|   stm32f427_437_429_439_lqfp176 IBIS Model
[IBIS ver]   4.2
[File name]  stm32f427_437_429_439_lqfp176.ibs
[File Rev]   1.3
[Date]   05-30-2014
[Source] Data Created at STMicroelectronics
[Notes]   File originated from ELDO simulations.
[Disclaimer]  This information is for modeling purpose only and is
   not guaranted. The information is subject to change without
   notice.
[Copyright] Copyright 2014 STMicroelectronics Inc.
[Component] stm32f427_437_429_439_lqfp176
[Manufacturer] STMicroelectronics
[Package]
| variable   typ   min   max
R_pkg   0.0   NA   NA
L_pkg   0.0H   NA   NA
C_pkg   0.0F   NA   NA
[Pin]   signal_name   model_name   R_pin   L_pin   C_pin
1   PE2   io8p_arsudq_ft   235.0E-3   11.5E-9   327.0E-15
2   PE3   io8p_arsudq_ft   229.9E-3   11.2E-9   303.3E-15
3   PE4   io8p_arsudq_ft   225.0E-3   10.8E-9   280.8E-15
4   PE5   io8p_arsudq_ft   220.4E-3   10.5E-9   259.5E-15
5   PE6   io8p_arsudq_ft   216.0E-3   10.3E-9   239.3E-15
6   VBAT   POWER   211.9E-3   10.0E-9   220.2E-15
7   PI8   io8p_arsudq_ft_v33   208.1E-3   9.7E-9   202.3E-15
8   PC13   io8p_arwsudq_ft_v33   204.4E-3   9.5E-9   185.6E-15
9   PC14   io8p_arwsudq_ft   201.1E-3   9.3E-9   170.0E-15
10   PC15   io8p_arsudq_ft   198.0E-3   9.1E-9   155.6E-15
11   PI9   io8p_arsudq_ft   195.1E-3   8.9E-9   142.3E-15
12   PI10   io8p_arsudq_ft   192.5E-3   8.7E-9   130.2E-15
13   PI11   io8p_arsudq_ft   190.1E-3   8.6E-9   119.2E-15
14   VSS   GND   188.0E-3   8.4E-9   109.4E-15
15   VDD   POWER   186.1E-3   8.3E-9   100.8E-15
16   PF0   io8p_arsudq_i2cin_ft   184.5E-3   8.2E-9   93.3E-15
17   PF1   io8p_arsudq_i2cin_ft   183.1E-3   8.1E-9   86.9E-15
18   PF2   io8p_arsudq_ft   182.0E-3   8.0E-9   81.7E-15
19   PF3   io8p_arwsudq_ft   181.1E-3   8.0E-9   77.7E-15
20   PF4   io8p_arwsudq_ft   180.5E-3   7.9E-9   74.8E-15
21   PF5   io8p_arwsudq_ft   180.1E-3   7.9E-9   73.1E-15
22   VSS   GND   180.0E-3   7.9E-9   72.5E-15
23   VDD   POWER   180.0E-3   7.9E-9   72.5E-15
24   PF6   io8p_arwsudq_ft   180.1E-3   7.9E-9   73.1E-15
25   PF7   io8p_arwsudq_ft   180.5E-3   7.9E-9   74.8E-15
26   PF8   io8p_arwsudq_ft   181.1E-3   8.0E-9   77.7E-15
27   PF9   io8p_arwsudq_ft   182.0E-3   8.0E-9   81.7E-15
28   PF10   io8p_arwsudq_ft   183.1E-3   8.1E-9   86.9E-15
29   PH0   io8p_arsudq_ft   184.5E-3   8.2E-9   93.3E-15
30   PH1   io8p_arsudq_ft   186.1E-3   8.3E-9   100.8E-15
31   NRST   ioreset_ft_v33   188.0E-3   8.4E-9   109.4E-15
32   PC0   io8p_ar3wsudq_ft   190.1E-3   8.6E-9   119.2E-15
33   PC1   io8p_ar3wsudq_ft   192.5E-3   8.7E-9   130.2E-15
34   PC2   io8p_ar3wsudq_ft   195.1E-3   8.9E-9   142.3E-15
35   PC3   io8p_ar3wsudq_ft   198.0E-3   9.1E-9   155.6E-15
36   VDD   POWER   201.1E-3   9.3E-9   170.0E-15
37   VREFM   POWER   204.4E-3   9.5E-9   185.6E-15
38   VREFP   POWER   208.1E-3   9.7E-9   202.3E-15
39   VDDA   POWER   211.9E-3   10.0E-9   220.2E-15
40   PA0   io8p_ar3wsudq_ft_v33   216.0E-3   10.3E-9   239.3E-15
41   PA1   io8p_ar3wsudq_ft   220.4E-3   10.5E-9   259.5E-15
42   PA2   io8p_ar3wsudq_ft   225.0E-3   10.8E-9   280.8E-15
43   PH2   io8p_arsudq_ft   229.9E-3   11.2E-9   303.3E-15
44   PH3   io8p_arsudq_ft   235.0E-3   11.5E-9   327.0E-15
45   PH4   io8p_arsudq_i2cin_ft   235.0E-3   11.5E-9   327.0E-15
46   PH5   io8p_arsudq_i2cin_ft   229.9E-3   11.2E-9   303.3E-15
47   PA3   io8p_ar3wsudq_ft   225.0E-3   10.8E-9   280.8E-15
48   BYPASS_REG   io8p_arsudq_ft_v33   220.4E-3   10.5E-9   259.5E-15
49   VDD   POWER   216.0E-3   10.3E-9   239.3E-15
50   PA4   io8p_ar3wsudq_ft   211.9E-3   10.0E-9   220.2E-15
51   PA5   io8p_ar3wsudq_ft   208.1E-3   9.7E-9   202.3E-15
52   PA6   io8p_ar3wsudq_ft   204.4E-3   9.5E-9   185.6E-15
53   PA7   io8p_ar3wsudq_ft   201.1E-3   9.3E-9   170.0E-15
54   PC4   io8p_ar3wsudq_ft   198.0E-3   9.1E-9   155.6E-15
55   PC5   io8p_ar3wsudq_ft   195.1E-3   8.9E-9   142.3E-15
56   PB0   io8p_ar3wsudq_ft   192.5E-3   8.7E-9   130.2E-15
57   PB1   io8p_ar3wsudq_ft   190.1E-3   8.6E-9   119.2E-15
58   PB2   io8p_ar3wsudq_ft   188.0E-3   8.4E-9   109.4E-15
59   PF11   io8p_arsudq_ft   186.1E-3   8.3E-9   100.8E-15
60   PF12   io8p_arsudq_ft   184.5E-3   8.2E-9   93.3E-15
61   VSS   GND   183.1E-3   8.1E-9   86.9E-15
62   VDD   POWER   182.0E-3   8.0E-9   81.7E-15
63   PF13   io8p_arsudq_ft   181.1E-3   8.0E-9   77.7E-15
64   PF14   io8p_arsudq_ft   180.5E-3   7.9E-9   74.8E-15
65   PF15   io8p_arsudq_ft   180.1E-3   7.9E-9   73.1E-15
66   PG0   io8p_arsudq_ft   180.0E-3   7.9E-9   72.5E-15
67   PG1   io8p_arsudq_ft   180.0E-3   7.9E-9   72.5E-15
68   PE7   io8p_arsudq_ft   180.1E-3   7.9E-9   73.1E-15
69   PE8   io8p_arsudq_ft   180.5E-3   7.9E-9   74.8E-15
70   PE9   io8p_arsudq_ft   181.1E-3   8.0E-9   77.7E-15
71   VSS   GND   182.0E-3   8.0E-9   81.7E-15
72   VDD   POWER   183.1E-3   8.1E-9   86.9E-15
73   PE10   io8p_arsudq_ft   184.5E-3   8.2E-9   93.3E-15
74   PE11   io8p_arsudq_ft   186.1E-3   8.3E-9   100.8E-15
75   PE12   io8p_arsudq_ft   188.0E-3   8.4E-9   109.4E-15
76   PE13   io8p_arsudq_ft   190.1E-3   8.6E-9   119.2E-15
77   PE14   io8p_arsudq_ft   192.5E-3   8.7E-9   130.2E-15
78   PE15   io8p_ar3wsudq_ft   195.1E-3   8.9E-9   142.3E-15
79   PB10   io8p_arsudq_i2cin_ft   198.0E-3   9.1E-9   155.6E-15
80   PB11   io8p_arsudq_i2cin_ft   201.1E-3   9.3E-9   170.0E-15
81   VCAP1   POWER   204.4E-3   9.5E-9   185.6E-15
82   VDD   POWER   208.1E-3   9.7E-9   202.3E-15
83   PH6   io8p_arsudq_ft   211.9E-3   10.0E-9   220.2E-15
84   PH7   io8p_arsudq_i2cin_ft   216.0E-3   10.3E-9   239.3E-15
85   PH8   io8p_arsudq_i2cin_ft   220.4E-3   10.5E-9   259.5E-15
86   PH9   io8p_arsudq_ft   225.0E-3   10.8E-9   280.8E-15
87   PH10   io8p_arsudq_ft   229.9E-3   11.2E-9   303.3E-15
88   PH11   io8p_arsudq_ft   235.0E-3   11.5E-9   327.0E-15
89   PH12   io8p_arsudq_ft   235.0E-3   11.5E-9   327.0E-15
90   VSS   GND   229.9E-3   11.2E-9   303.3E-15
91   VDD   POWER   225.0E-3   10.8E-9   280.8E-15
92   PB12   io8usb_id_otg_ft   220.4E-3   10.5E-9   259.5E-15
93   PB13   io8usb_vbus_otg_ft   216.0E-3   10.3E-9   239.3E-15
94   PB14   io8usb_lsfs_otg_ft   211.9E-3   10.0E-9   220.2E-15
95   PB15   io8usb_lsfs_otg_ft   208.1E-3   9.7E-9   202.3E-15
96   PD8   io8p_arsudq_ft   204.4E-3   9.5E-9   185.6E-15
97   PD9   io8p_arsudq_ft   201.1E-3   9.3E-9   170.0E-15
98   PD10   io8p_arsudq_ft   198.0E-3   9.1E-9   155.6E-15
99   PD11   io8p_arsudq_ft   195.1E-3   8.9E-9   142.3E-15
100   PD12   io8p_arsudq_ft   192.5E-3   8.7E-9   130.2E-15
101   PD13   io8p_arsudq_ft   190.1E-3   8.6E-9   119.2E-15
102   VSS   GND   188.0E-3   8.4E-9   109.4E-15
103   VDD   POWER   186.1E-3   8.3E-9   100.8E-15
104   PD14   io8p_arsudq_ft   184.5E-3   8.2E-9   93.3E-15
105   PD15   io8p_arsudq_ft   183.1E-3   8.1E-9   86.9E-15
106   PG2   io8p_arsudq_ft   182.0E-3   8.0E-9   81.7E-15
107   PG3   io8p_arsudq_ft   181.1E-3   8.0E-9   77.7E-15
108   PG4   io8p_arsudq_ft   180.5E-3   7.9E-9   74.8E-15
109   PG5   io8p_arsudq_ft   180.1E-3   7.9E-9   73.1E-15
110   PG6   io8p_arsudq_ft   180.0E-3   7.9E-9   72.5E-15
111   PG7   io8p_arsudq_ft   180.0E-3   7.9E-9   72.5E-15
112   PG8   io8p_arsudq_ft   180.1E-3   7.9E-9   73.1E-15
113   VSS   GND   180.5E-3   7.9E-9   74.8E-15
114   VDD   POWER   181.1E-3   8.0E-9   77.7E-15
115   PC6   io8p_arsudq_ft   182.0E-3   8.0E-9   81.7E-15
116   PC7   io8p_arsudq_ft   183.1E-3   8.1E-9   86.9E-15
117   PC8   io8p_arsudq_ft   184.5E-3   8.2E-9   93.3E-15
118   PC9   io8p_arsudq_i2cin_ft   186.1E-3   8.3E-9   100.8E-15
119   PA8   io8p_arsudq_i2cin_ft   188.0E-3   8.4E-9   109.4E-15
120   PA9   io8usb_vbus_otg_ft   190.1E-3   8.6E-9   119.2E-15
121   PA10   io8usb_id_otg_ft   192.5E-3   8.7E-9   130.2E-15
122   PA11   io8usb_lsfs_otg_ft   195.1E-3   8.9E-9   142.3E-15
123   PA12   io8usb_lsfs_otg_ft   198.0E-3   9.1E-9   155.6E-15
124   PA13   io8p_arsudq_ft   201.1E-3   9.3E-9   170.0E-15
125   VCAP2   POWER   204.4E-3   9.5E-9   185.6E-15
126   VSS   GND   208.1E-3   9.7E-9   202.3E-15
127   VDD   POWER   211.9E-3   10.0E-9   220.2E-15
128   PH13   io8p_arsudq_ft   216.0E-3   10.3E-9   239.3E-15
129   PH14   io8p_arsudq_ft   220.4E-3   10.5E-9   259.5E-15
130   PH15   io8p_arsudq_ft   225.0E-3   10.8E-9   280.8E-15
131   PI0   io8p_arsudq_ft   229.9E-3   11.2E-9   303.3E-15
132   PI1   io8p_arsudq_ft   235.0E-3   11.5E-9   327.0E-15
133   PI2   io8p_arsudq_ft   235.0E-3   11.5E-9   327.0E-15
134   PI3   io8p_arsudq_ft   229.9E-3   11.2E-9   303.3E-15
135   VSS   GND   225.0E-3   10.8E-9   280.8E-15
136   VDD   POWER   220.4E-3   10.5E-9   259.5E-15
137   PA14   io8p_arsudq_ft   216.0E-3   10.3E-9   239.3E-15
138   PA15   io8p_arsudq_ft   211.9E-3   10.0E-9   220.2E-15
139   PC10   io8p_arsudq_ft   208.1E-3   9.7E-9   202.3E-15
140   PC11   io8p_arsudq_ft   204.4E-3   9.5E-9   185.6E-15
141   PC12   io8p_arsudq_ft   201.1E-3   9.3E-9   170.0E-15
142   PD0   io8p_arsudq_ft   198.0E-3   9.1E-9   155.6E-15
143   PD1   io8p_arsudq_ft   195.1E-3   8.9E-9   142.3E-15
144   PD2   io8p_arsudq_ft   192.5E-3   8.7E-9   130.2E-15
145   PD3   io8p_arsudq_ft   190.1E-3   8.6E-9   119.2E-15
146   PD4   io8p_arsudq_ft   188.0E-3   8.4E-9   109.4E-15
147   PD5   io8p_arsudq_ft   186.1E-3   8.3E-9   100.8E-15
148   VSS   GND   184.5E-3   8.2E-9   93.3E-15
149   VDD   POWER   183.1E-3   8.1E-9   86.9E-15
150   PD6   io8p_arsudq_ft   182.0E-3   8.0E-9   81.7E-15
151   PD7   io8p_arsudq_ft   181.1E-3   8.0E-9   77.7E-15
152   PG9   io8p_arsudq_ft   180.5E-3   7.9E-9   74.8E-15
153   PG10   io8p_arsudq_ft   180.1E-3   7.9E-9   73.1E-15
154   PG11   io8p_arsudq_ft   180.0E-3   7.9E-9   72.5E-15
155   PG12   io8p_arsudq_ft   180.0E-3   7.9E-9   72.5E-15
156   PG13   io8p_arsudq_ft   180.1E-3   7.9E-9   73.1E-15
157   PG14   io8p_arsudq_ft   180.5E-3   7.9E-9   74.8E-15
158   VSS   GND   181.1E-3   8.0E-9   77.7E-15
159   VDD   POWER   182.0E-3   8.0E-9   81.7E-15
160   PG15   io8p_arsudq_ft   183.1E-3   8.1E-9   86.9E-15
161   PB3   io8p_arsudq_ft   184.5E-3   8.2E-9   93.3E-15
162   PB4   io8p_arsudq_ft   186.1E-3   8.3E-9   100.8E-15
163   PB5   io8p_ar3wsudq_ft   188.0E-3   8.4E-9   109.4E-15
164   PB6   io8p_arsudq_i2cin_ft   190.1E-3   8.6E-9   119.2E-15
165   PB7   io8p_arsudq_i2cin_ft   192.5E-3   8.7E-9   130.2E-15
166   BOOT0   vpp_test_hv   195.1E-3   8.9E-9   142.3E-15
167   PB8   io8p_arsudq_i2cin_ft   198.0E-3   9.1E-9   155.6E-15
168   PB9   io8p_arsudq_i2cin_ft   201.1E-3   9.3E-9   170.0E-15
169   PE0   io8p_arsudq_ft   204.4E-3   9.5E-9   185.6E-15
170   PE1   io8p_arsudq_ft   208.1E-3   9.7E-9   202.3E-15
171   PDR_ON   io8p_arsudq_ft_v33   211.9E-3   10.0E-9   220.2E-15
172   VDD_3   POWER   216.0E-3   10.3E-9   239.3E-15
173   PI4   io8p_arsudq_ft   220.4E-3   10.5E-9   259.5E-15
174   PI5   io8p_arsudq_ft   225.0E-3   10.8E-9   280.8E-15
175   PI6   io8p_arsudq_ft   229.9E-3   11.2E-9   303.3E-15
176   PI7   io8p_arsudq_ft   235.0E-3   11.5E-9   327.0E-15
[Diff Pin]   inv_pin   vdiff   tdelay_typ  tdelay_min  tdelay_max
95   94   200mV   NA   NA   NA
123   122   200mV   NA   NA   NA
[Model Selector] io8p_ar3wsudq_ft
io8p00_ar3wsudq_ft_pd_lv  "SPEED00 1P8V, PD=40kOhm"
io8p00_ar3wsudq_ft_pu_lv  "SPEED00 1P8V, PU=40kOhm"
io8p00_ar3wsudq_ft_lv  "SPEED00 1P8V"
io8p01_ar3wsudq_ft_pd_lv  "SPEED01 1P8V, PD=40kOhm"
io8p01_ar3wsudq_ft_pu_lv  "SPEED01 1P8V, PU=40kOhm"
io8p01_ar3wsudq_ft_lv  "SPEED01 1P8V"
io8p10_ar3wsudq_ft_pd_lv  "SPEED10 1P8V, PD=40kOhm"
io8p10_ar3wsudq_ft_pu_lv  "SPEED10 1P8V, PU=40kOhm"
io8p10_ar3wsudq_ft_lv  "SPEED10 1P8V"
io8p11_ar3wsudq_ft_pd_lv  "SPEED11 1P8V, PD=40kOhm"
io8p11_ar3wsudq_ft_pu_lv  "SPEED11 1P8V, PU=40kOhm"
io8p11_ar3wsudq_ft_lv  "SPEED11 1P8V"
io8p00_ar3wsudq_ft_pd  "SPEED00, PD=40kOhm"
io8p00_ar3wsudq_ft_pu  "SPEED00, PU=40kOhm"
io8p00_ar3wsudq_ft  "SPEED00"
io8p01_ar3wsudq_ft_pd  "SPEED01, PD=40kOhm"
io8p01_ar3wsudq_ft_pu  "SPEED01, PU=40kOhm"
io8p01_ar3wsudq_ft  "SPEED01"
io8p10_ar3wsudq_ft_pd  "SPEED10, PD=40kOhm"
io8p10_ar3wsudq_ft_pu  "SPEED10, PU=40kOhm"
io8p10_ar3wsudq_ft  "SPEED10"
io8p11_ar3wsudq_ft_pd  "SPEED11, PD=40kOhm"
io8p11_ar3wsudq_ft_pu  "SPEED11, PU=40kOhm"
io8p11_ar3wsudq_ft  "SPEED11"
[Model Selector] io8p_ar3wsudq_ft_v33
io8p00_ar3wsudq_ft_v33_pd_lv  "SPEED00 1P8V, PD=40kOhm"
io8p00_ar3wsudq_ft_v33_pu_lv  "SPEED00 1P8V, PU=40kOhm"
io8p00_ar3wsudq_ft_v33_lv  "SPEED00 1P8V"
io8p01_ar3wsudq_ft_v33_pd_lv  "SPEED01 1P8V, PD=40kOhm"
io8p01_ar3wsudq_ft_v33_pu_lv  "SPEED01 1P8V, PU=40kOhm"
io8p01_ar3wsudq_ft_v33_lv  "SPEED01 1P8V"
io8p10_ar3wsudq_ft_v33_pd_lv  "SPEED10 1P8V, PD=40kOhm"
io8p10_ar3wsudq_ft_v33_pu_lv  "SPEED10 1P8V, PU=40kOhm"
io8p10_ar3wsudq_ft_v33_lv  "SPEED10 1P8V"
io8p11_ar3wsudq_ft_v33_pd_lv  "SPEED11 1P8V, PD=40kOhm"
io8p11_ar3wsudq_ft_v33_pu_lv  "SPEED11 1P8V, PU=40kOhm"
io8p11_ar3wsudq_ft_v33_lv  "SPEED11 1P8V"
io8p00_ar3wsudq_ft_v33_pd  "SPEED00, PD=40kOhm"
io8p00_ar3wsudq_ft_v33_pu  "SPEED00, PU=40kOhm"
io8p00_ar3wsudq_ft_v33  "SPEED00"
io8p01_ar3wsudq_ft_v33_pd  "SPEED01, PD=40kOhm"
io8p01_ar3wsudq_ft_v33_pu  "SPEED01, PU=40kOhm"
io8p01_ar3wsudq_ft_v33  "SPEED01"
io8p10_ar3wsudq_ft_v33_pd  "SPEED10, PD=40kOhm"
io8p10_ar3wsudq_ft_v33_pu  "SPEED10, PU=40kOhm"
io8p10_ar3wsudq_ft_v33  "SPEED10"
io8p11_ar3wsudq_ft_v33_pd  "SPEED11, PD=40kOhm"
io8p11_ar3wsudq_ft_v33_pu  "SPEED11, PU=40kOhm"
io8p11_ar3wsudq_ft_v33  "SPEED11"
[Model Selector] io8p_arsudq_ft
io8p00_arsudq_ft_pd_lv  "SPEED00 1P8V, PD=40kOhm"
io8p00_arsudq_ft_pu_lv  "SPEED00 1P8V, PU=40kOhm"
io8p00_arsudq_ft_lv  "SPEED00 1P8V"
io8p01_arsudq_ft_pd_lv  "SPEED01 1P8V, PD=40kOhm"
io8p01_arsudq_ft_pu_lv  "SPEED01 1P8V, PU=40kOhm"
io8p01_arsudq_ft_lv  "SPEED01 1P8V"
io8p10_arsudq_ft_pd_lv  "SPEED10 1P8V, PD=40kOhm"
io8p10_arsudq_ft_pu_lv  "SPEED10 1P8V, PU=40kOhm"
io8p10_arsudq_ft_lv  "SPEED10 1P8V"
io8p11_arsudq_ft_pd_lv  "SPEED11 1P8V, PD=40kOhm"
io8p11_arsudq_ft_pu_lv  "SPEED11 1P8V, PU=40kOhm"
io8p11_arsudq_ft_lv  "SPEED11 1P8V"
io8p00_arsudq_ft_pd  "SPEED00, PD=40kOhm"
io8p00_arsudq_ft_pu  "SPEED00, PU=40kOhm"
io8p00_arsudq_ft  "SPEED00"
io8p01_arsudq_ft_pd  "SPEED01, PD=40kOhm"
io8p01_arsudq_ft_pu  "SPEED01, PU=40kOhm"
io8p01_arsudq_ft  "SPEED01"
io8p10_arsudq_ft_pd  "SPEED10, PD=40kOhm"
io8p10_arsudq_ft_pu  "SPEED10, PU=40kOhm"
io8p10_arsudq_ft  "SPEED10"
io8p11_arsudq_ft_pd  "SPEED11, PD=40kOhm"
io8p11_arsudq_ft_pu  "SPEED11, PU=40kOhm"
io8p11_arsudq_ft  "SPEED11"
[Model Selector] io8p_arsudq_ft_v33
io8p00_arsudq_ft_v33_pd_lv  "SPEED00 1P8V, PD=40kOhm"
io8p00_arsudq_ft_v33_pu_lv  "SPEED00 1P8V, PU=40kOhm"
io8p00_arsudq_ft_v33_lv  "SPEED00 1P8V"
io8p01_arsudq_ft_v33_pd_lv  "SPEED01 1P8V, PD=40kOhm"
io8p01_arsudq_ft_v33_pu_lv  "SPEED01 1P8V, PU=40kOhm"
io8p01_arsudq_ft_v33_lv  "SPEED01 1P8V"
io8p10_arsudq_ft_v33_pd_lv  "SPEED10 1P8V, PD=40kOhm"
io8p10_arsudq_ft_v33_pu_lv  "SPEED10 1P8V, PU=40kOhm"
io8p10_arsudq_ft_v33_lv  "SPEED10 1P8V"
io8p11_arsudq_ft_v33_pd_lv  "SPEED11 1P8V, PD=40kOhm"
io8p11_arsudq_ft_v33_pu_lv  "SPEED11 1P8V, PU=40kOhm"
io8p11_arsudq_ft_v33_lv  "SPEED11 1P8V"
io8p00_arsudq_ft_v33_pd  "SPEED00, PD=40kOhm"
io8p00_arsudq_ft_v33_pu  "SPEED00, PU=40kOhm"
io8p00_arsudq_ft_v33  "SPEED00"
io8p01_arsudq_ft_v33_pd  "SPEED01, PD=40kOhm"
io8p01_arsudq_ft_v33_pu  "SPEED01, PU=40kOhm"
io8p01_arsudq_ft_v33  "SPEED01"
io8p10_arsudq_ft_v33_pd  "SPEED10, PD=40kOhm"
io8p10_arsudq_ft_v33_pu  "SPEED10, PU=40kOhm"
io8p10_arsudq_ft_v33  "SPEED10"
io8p11_arsudq_ft_v33_pd  "SPEED11, PD=40kOhm"
io8p11_arsudq_ft_v33_pu  "SPEED11, PU=40kOhm"
io8p11_arsudq_ft_v33  "SPEED11"
[Model Selector] io8p_arsudq_i2cin_ft
io8p00_arsudq_i2cin_ft_pd_lv  "SPEED00 1P8V, PD=40kOhm"
io8p00_arsudq_i2cin_ft_pu_lv  "SPEED00 1P8V, PU=40kOhm"
io8p00_arsudq_i2cin_ft_lv  "SPEED00 1P8V"
io8p01_arsudq_i2cin_ft_pd_lv  "SPEED01 1P8V, PD=40kOhm"
io8p01_arsudq_i2cin_ft_pu_lv  "SPEED01 1P8V, PU=40kOhm"
io8p01_arsudq_i2cin_ft_lv  "SPEED01 1P8V"
io8p10_arsudq_i2cin_ft_pd_lv  "SPEED10 1P8V, PD=40kOhm"
io8p10_arsudq_i2cin_ft_pu_lv  "SPEED10 1P8V, PU=40kOhm"
io8p10_arsudq_i2cin_ft_lv  "SPEED10 1P8V"
io8p11_arsudq_i2cin_ft_pd_lv  "SPEED11 1P8V, PD=40kOhm"
io8p11_arsudq_i2cin_ft_pu_lv  "SPEED11 1P8V, PU=40kOhm"
io8p11_arsudq_i2cin_ft_lv  "SPEED11 1P8V"
io8p00_arsudq_i2cin_ft_pd  "SPEED00, PD=40kOhm"
io8p00_arsudq_i2cin_ft_pu  "SPEED00, PU=40kOhm"
io8p00_arsudq_i2cin_ft  "SPEED00"
io8p01_arsudq_i2cin_ft_pd  "SPEED01, PD=40kOhm"
io8p01_arsudq_i2cin_ft_pu  "SPEED01, PU=40kOhm"
io8p01_arsudq_i2cin_ft  "SPEED01"
io8p10_arsudq_i2cin_ft_pd  "SPEED10, PD=40kOhm"
io8p10_arsudq_i2cin_ft_pu  "SPEED10, PU=40kOhm"
io8p10_arsudq_i2cin_ft  "SPEED10"
io8p11_arsudq_i2cin_ft_pd  "SPEED11, PD=40kOhm"
io8p11_arsudq_i2cin_ft_pu  "SPEED11, PU=40kOhm"
io8p11_arsudq_i2cin_ft  "SPEED11"
[Model Selector] io8p_arwsudq_ft
io8p00_arwsudq_ft_pd_lv  "SPEED00 1P8V, PD=40kOhm"
io8p00_arwsudq_ft_pu_lv  "SPEED00 1P8V, PU=40kOhm"
io8p00_arwsudq_ft_lv  "SPEED00 1P8V"
io8p01_arwsudq_ft_pd_lv  "SPEED01 1P8V, PD=40kOhm"
io8p01_arwsudq_ft_pu_lv  "SPEED01 1P8V, PU=40kOhm"
io8p01_arwsudq_ft_lv  "SPEED01 1P8V"
io8p10_arwsudq_ft_pd_lv  "SPEED10 1P8V, PD=40kOhm"
io8p10_arwsudq_ft_pu_lv  "SPEED10 1P8V, PU=40kOhm"
io8p10_arwsudq_ft_lv  "SPEED10 1P8V"
io8p11_arwsudq_ft_pd_lv  "SPEED11 1P8V, PD=40kOhm"
io8p11_arwsudq_ft_pu_lv  "SPEED11 1P8V, PU=40kOhm"
io8p11_arwsudq_ft_lv  "SPEED11 1P8V"
io8p00_arwsudq_ft_pd  "SPEED00, PD=40kOhm"
io8p00_arwsudq_ft_pu  "SPEED00, PU=40kOhm"
io8p00_arwsudq_ft  "SPEED00"
io8p01_arwsudq_ft_pd  "SPEED01, PD=40kOhm"
io8p01_arwsudq_ft_pu  "SPEED01, PU=40kOhm"
io8p01_arwsudq_ft  "SPEED01"
io8p10_arwsudq_ft_pd  "SPEED10, PD=40kOhm"
io8p10_arwsudq_ft_pu  "SPEED10, PU=40kOhm"
io8p10_arwsudq_ft  "SPEED10"
io8p11_arwsudq_ft_pd  "SPEED11, PD=40kOhm"
io8p11_arwsudq_ft_pu  "SPEED11, PU=40kOhm"
io8p11_arwsudq_ft  "SPEED11"
[Model Selector] io8p_arwsudq_ft_v33
io8p00_arwsudq_ft_v33_pd_lv  "SPEED00 1P8V, PD=40kOhm"
io8p00_arwsudq_ft_v33_pu_lv  "SPEED00 1P8V, PU=40kOhm"
io8p00_arwsudq_ft_v33_lv  "SPEED00 1P8V"
io8p01_arwsudq_ft_v33_pd_lv  "SPEED01 1P8V, PD=40kOhm"
io8p01_arwsudq_ft_v33_pu_lv  "SPEED01 1P8V, PU=40kOhm"
io8p01_arwsudq_ft_v33_lv  "SPEED01 1P8V"
io8p10_arwsudq_ft_v33_pd_lv  "SPEED10 1P8V, PD=40kOhm"
io8p10_arwsudq_ft_v33_pu_lv  "SPEED10 1P8V, PU=40kOhm"
io8p10_arwsudq_ft_v33_lv  "SPEED10 1P8V"
io8p11_arwsudq_ft_v33_pd_lv  "SPEED11 1P8V, PD=40kOhm"
io8p11_arwsudq_ft_v33_pu_lv  "SPEED11 1P8V, PU=40kOhm"
io8p11_arwsudq_ft_v33_lv  "SPEED11 1P8V"
io8p00_arwsudq_ft_v33_pd  "SPEED00, PD=40kOhm"
io8p00_arwsudq_ft_v33_pu  "SPEED00, PU=40kOhm"
io8p00_arwsudq_ft_v33  "SPEED00"
io8p01_arwsudq_ft_v33_pd  "SPEED01, PD=40kOhm"
io8p01_arwsudq_ft_v33_pu  "SPEED01, PU=40kOhm"
io8p01_arwsudq_ft_v33  "SPEED01"
io8p10_arwsudq_ft_v33_pd  "SPEED10, PD=40kOhm"
io8p10_arwsudq_ft_v33_pu  "SPEED10, PU=40kOhm"
io8p10_arwsudq_ft_v33  "SPEED10"
io8p11_arwsudq_ft_v33_pd  "SPEED11, PD=40kOhm"
io8p11_arwsudq_ft_v33_pu  "SPEED11, PU=40kOhm"
io8p11_arwsudq_ft_v33  "SPEED11"
[Model Selector] io8usb_id_otg_ft
io8p00_id_otg_ft_pd_lv  "SPEED00 1P8V, PD=14kOhm"
io8p00_id_otg_ft_pu_lv  "SPEED00 1P8V, PU=14kOhm"
io8p00_id_otg_ft_lv  "SPEED00 1P8V"
io8p01_id_otg_ft_pd_lv  "SPEED01 1P8V, PD=14kOhm"
io8p01_id_otg_ft_pu_lv  "SPEED01 1P8V, PU=14kOhm"
io8p01_id_otg_ft_lv  "SPEED01 1P8V"
io8p10_id_otg_ft_pd_lv  "SPEED10 1P8V, PD=14kOhm"
io8p10_id_otg_ft_pu_lv  "SPEED10 1P8V, PU=14kOhm"
io8p10_id_otg_ft_lv  "SPEED10 1P8V"
io8p11_id_otg_ft_pd_lv  "SPEED11 1P8V, PD=14kOhm"
io8p11_id_otg_ft_pu_lv  "SPEED11 1P8V, PU=14kOhm"
io8p11_id_otg_ft_lv  "SPEED11 1P8V"
io8p00_id_otg_ft_pd  "SPEED00, PD=14kOhm"
io8p00_id_otg_ft_pu  "SPEED00, PU=14kOhm"
io8p00_id_otg_ft  "SPEED00"
io8p01_id_otg_ft_pd  "SPEED01, PD=14kOhm"
io8p01_id_otg_ft_pu  "SPEED01, PU=14kOhm"
io8p01_id_otg_ft  "SPEED01"
io8p10_id_otg_ft_pd  "SPEED10, PD=14kOhm"
io8p10_id_otg_ft_pu  "SPEED10, PU=14kOhm"
io8p10_id_otg_ft  "SPEED10"
io8p11_id_otg_ft_pd  "SPEED11, PD=14kOhm"
io8p11_id_otg_ft_pu  "SPEED11, PU=14kOhm"
io8p11_id_otg_ft  "SPEED11"
[Model Selector] io8usb_lsfs_otg_ft
io8usb_ls_otg_ft_dpdn_pd  "LS USB DP/DN IO + PD=20kOhm"
io8usb_ls_otg_ft_dpdn_pupu2  "LS USB DP/DN IO + PU/PU2=2.2kOhm"
io8usb_ls_otg_ft_dpdn_pu2  "LS USB DP/DN IO + PU2=1.2kOhm"
io8usb_ls_otg_ft_dpdn_pu  "LS USB DP/DN IO + PU=1.2kOhm"
io8usb_ls_otg_ft_dpdn  "LS USB DP/DN IO"
io8usb_fs_otg_ft_dpdn_pd  "HS USB DP/DN IO + PD=20kOhm"
io8usb_fs_otg_ft_dpdn_pupu2  "HS USB DP/DN IO + PU/PU2=2.2kOhm"
io8usb_fs_otg_ft_dpdn_pu2  "HS USB DP/DN IO + PU2=1.2kOhm"
io8usb_fs_otg_ft_dpdn_pu  "HS USB DP/DN IO + PU=1.2kOhm"
io8usb_fs_otg_ft_dpdn  "HS USB DP/DN IO"
io8p00_lsfs_otg_ft_pd_lv  "SPEED00 1P8V, PD=40kOhm"
io8p00_lsfs_otg_ft_pu_lv  "SPEED00 1P8V, PU=40kOhm"
io8p00_lsfs_otg_ft_lv  "SPEED00 1P8V"
io8p01_lsfs_otg_ft_pd_lv  "SPEED01 1P8V, PD=40kOhm"
io8p01_lsfs_otg_ft_pu_lv  "SPEED01 1P8V, PU=40kOhm"
io8p01_lsfs_otg_ft_lv  "SPEED01 1P8V"
io8p10_lsfs_otg_ft_pd_lv  "SPEED10 1P8V, PD=40kOhm"
io8p10_lsfs_otg_ft_pu_lv  "SPEED10 1P8V, PU=40kOhm"
io8p10_lsfs_otg_ft_lv  "SPEED10 1P8V"
io8p11_lsfs_otg_ft_pd_lv  "SPEED11 1P8V, PD=40kOhm"
io8p11_lsfs_otg_ft_pu_lv  "SPEED11 1P8V, PU=40kOhm"
io8p11_lsfs_otg_ft_lv  "SPEED11 1P8V"
io8p00_lsfs_otg_ft_pd  "SPEED00, PD=40kOhm"
io8p00_lsfs_otg_ft_pu  "SPEED00, PU=40kOhm"
io8p00_lsfs_otg_ft  "SPEED00"
io8p01_lsfs_otg_ft_pd  "SPEED01, PD=40kOhm"
io8p01_lsfs_otg_ft_pu  "SPEED01, PU=40kOhm"
io8p01_lsfs_otg_ft  "SPEED01"
io8p10_lsfs_otg_ft_pd  "SPEED10, PD=40kOhm"
io8p10_lsfs_otg_ft_pu  "SPEED10, PU=40kOhm"
io8p10_lsfs_otg_ft  "SPEED10"
io8p11_lsfs_otg_ft_pd  "SPEED11, PD=40kOhm"
io8p11_lsfs_otg_ft_pu  "SPEED11, PU=40kOhm"
io8p11_lsfs_otg_ft  "SPEED11"
[Model Selector] io8usb_vbus_otg_ft
io8psenb_vbus_otg_ft  "VBUS PULSE, SENSE VB"
io8psenab_vbus_otg_ft  "VBUS PULSE, SENSE VA and VB"
io8psena_vbus_otg_ft  "VBUS PULSE, SENSE VA"
io8psen_vbus_otg_ft  "VBUS PULSE"
io8p00_vbus_otg_ft_pd_lv  "SPEED00 1P8V, PD=40kOhm"
io8p00_vbus_otg_ft_pu_lv  "SPEED00 1P8V, PU=40kOhm"
io8p00_vbus_otg_ft_lv  "SPEED00 1P8V"
io8p01_vbus_otg_ft_pd_lv  "SPEED01 1P8V, PD=40kOhm"
io8p01_vbus_otg_ft_pu_lv  "SPEED01 1P8V, PU=40kOhm"
io8p01_vbus_otg_ft_lv  "SPEED01 1P8V"
io8p10_vbus_otg_ft_pd_lv  "SPEED10 1P8V, PD=40kOhm"
io8p10_vbus_otg_ft_pu_lv  "SPEED10 1P8V, PU=40kOhm"
io8p10_vbus_otg_ft_lv  "SPEED10 1P8V"
io8p11_vbus_otg_ft_pd_lv  "SPEED11 1P8V, PD=40kOhm"
io8p11_vbus_otg_ft_pu_lv  "SPEED11 1P8V, PU=40kOhm"
io8p11_vbus_otg_ft_lv  "SPEED11 1P8V"
io8p00_vbus_otg_ft_pd  "SPEED00, PD=40kOhm"
io8p00_vbus_otg_ft_pu  "SPEED00, PU=40kOhm"
io8p00_vbus_otg_ft  "SPEED00"
io8p01_vbus_otg_ft_pd  "SPEED01, PD=40kOhm"
io8p01_vbus_otg_ft_pu  "SPEED01, PU=40kOhm"
io8p01_vbus_otg_ft  "SPEED01"
io8p10_vbus_otg_ft_pd  "SPEED10, PD=40kOhm"
io8p10_vbus_otg_ft_pu  "SPEED10, PU=40kOhm"
io8p10_vbus_otg_ft  "SPEED10"
io8p11_vbus_otg_ft_pd  "SPEED11, PD=40kOhm"
io8p11_vbus_otg_ft_pu  "SPEED11, PU=40kOhm"
io8p11_vbus_otg_ft  "SPEED11"
[Model Selector] ioreset_ft_v33
ioreset_ft_v33_pu_lv  "ioreset 1P8V + PU=40kOhm"
ioreset_ft_v33_nopu_lv  "ioreset 1P8V"
ioreset_ft_v33_pu  "ioreset + PU=40kOhm"
ioreset_ft_v33_nopu  "ioreset"
[Model Selector] vpp_test_hv
vpp_test_hv_2p4  "Input Buffer 1P8V"
vpp_test_hv_3p3  "Input Buffer"
| Models and submodels in the file (260): io8p00_ar3wsudq_ft_pd_lv (I/O), io8p00_ar3wsudq_ft_pu_lv (I/O), io8p00_ar3wsudq_ft_lv (I/O), io8p01_ar3wsudq_ft_pd_lv (I/O), io8p01_ar3wsudq_ft_pu_lv (I/O), io8p01_ar3wsudq_ft_lv (I/O), io8p10_ar3wsudq_ft_pd_lv (I/O), io8p10_ar3wsudq_ft_pu_lv (I/O), io8p10_ar3wsudq_ft_lv (I/O), io8p11_ar3wsudq_ft_pd_lv (I/O), io8p11_ar3wsudq_ft_pu_lv (I/O), io8p11_ar3wsudq_ft_lv (I/O), io8p00_ar3wsudq_ft_pd (I/O), io8p00_ar3wsudq_ft_pu (I/O), io8p00_ar3wsudq_ft (I/O), io8p01_ar3wsudq_ft_pd (I/O), io8p01_ar3wsudq_ft_pu (I/O), io8p01_ar3wsudq_ft (I/O), io8p10_ar3wsudq_ft_pd (I/O), io8p10_ar3wsudq_ft_pu (I/O), io8p10_ar3wsudq_ft (I/O), io8p11_ar3wsudq_ft_pd (I/O), io8p11_ar3wsudq_ft_pu (I/O), io8p11_ar3wsudq_ft (I/O), io8p00_ar3wsudq_ft_v33_pd_lv (I/O), io8p00_ar3wsudq_ft_v33_pu_lv (I/O), io8p00_ar3wsudq_ft_v33_lv (I/O), io8p01_ar3wsudq_ft_v33_pd_lv (I/O), io8p01_ar3wsudq_ft_v33_pu_lv (I/O), io8p01_ar3wsudq_ft_v33_lv (I/O), io8p10_ar3wsudq_ft_v33_pd_lv (I/O), io8p10_ar3wsudq_ft_v33_pu_lv (I/O), io8p10_ar3wsudq_ft_v33_lv (I/O), io8p11_ar3wsudq_ft_v33_pd_lv (I/O), io8p11_ar3wsudq_ft_v33_pu_lv (I/O), io8p11_ar3wsudq_ft_v33_lv (I/O), io8p00_ar3wsudq_ft_v33_pd (I/O), io8p00_ar3wsudq_ft_v33_pu (I/O), io8p00_ar3wsudq_ft_v33 (I/O), io8p01_ar3wsudq_ft_v33_pd (I/O), io8p01_ar3wsudq_ft_v33_pu (I/O), io8p01_ar3wsudq_ft_v33 (I/O), io8p10_ar3wsudq_ft_v33_pd (I/O), io8p10_ar3wsudq_ft_v33_pu (I/O), io8p10_ar3wsudq_ft_v33 (I/O), io8p11_ar3wsudq_ft_v33_pd (I/O), io8p11_ar3wsudq_ft_v33_pu (I/O), io8p11_ar3wsudq_ft_v33 (I/O), io8p00_arsudq_ft_pd_lv (I/O), io8p00_arsudq_ft_pu_lv (I/O), io8p00_arsudq_ft_lv (I/O), io8p01_arsudq_ft_pd_lv (I/O), io8p01_arsudq_ft_pu_lv (I/O), io8p01_arsudq_ft_lv (I/O), io8p10_arsudq_ft_pd_lv (I/O), io8p10_arsudq_ft_pu_lv (I/O), io8p10_arsudq_ft_lv (I/O), io8p11_arsudq_ft_pd_lv (I/O), io8p11_arsudq_ft_pu_lv (I/O), io8p11_arsudq_ft_lv (I/O), io8p00_arsudq_ft_pd (I/O), io8p00_arsudq_ft_pu (I/O), io8p00_arsudq_ft (I/O), io8p01_arsudq_ft_pd (I/O), io8p01_arsudq_ft_pu (I/O), io8p01_arsudq_ft (I/O), io8p10_arsudq_ft_pd (I/O), io8p10_arsudq_ft_pu (I/O), io8p10_arsudq_ft (I/O), io8p11_arsudq_ft_pd (I/O), io8p11_arsudq_ft_pu (I/O), io8p11_arsudq_ft (I/O), io8p00_arsudq_ft_v33_pd_lv (I/O), io8p00_arsudq_ft_v33_pu_lv (I/O), io8p00_arsudq_ft_v33_lv (I/O), io8p01_arsudq_ft_v33_pd_lv (I/O), io8p01_arsudq_ft_v33_pu_lv (I/O), io8p01_arsudq_ft_v33_lv (I/O), io8p10_arsudq_ft_v33_pd_lv (I/O), io8p10_arsudq_ft_v33_pu_lv (I/O)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
